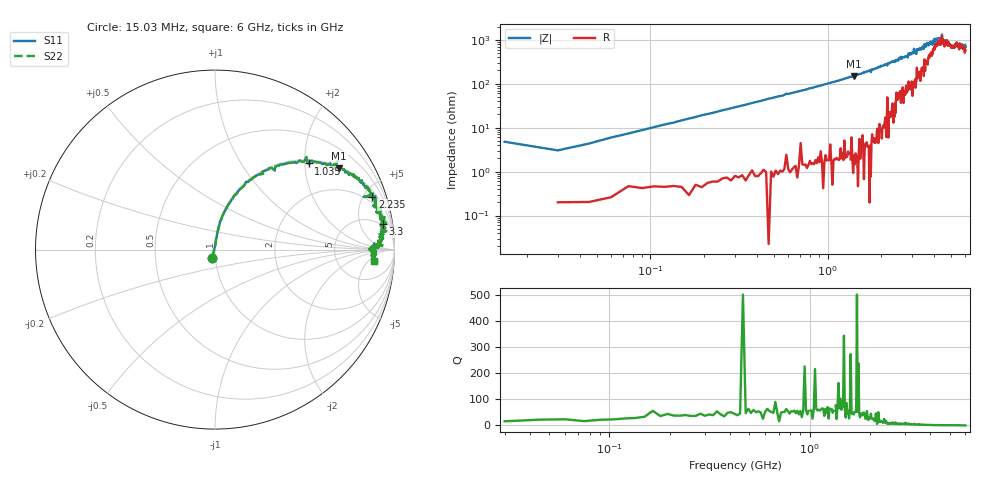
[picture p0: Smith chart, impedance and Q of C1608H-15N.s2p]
!	Network	Analyzer	HP8753E.07.74:	Oct	30	2002	Serial	No.	JP38451487
!	Hewlett-Packard
!	7	Sep	2009	10:19:27
!	Frequency	S11	S21	S12	S22
#	HZ	S	RI	R	50
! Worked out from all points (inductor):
!   400 points, 15.03 MHz to 6 GHz, reference 50 ohm
!   read as one part in series: L = 15.6 nH near 45.03 MHz
!   highest Q = 72 at 1.41 GHz (marker M1), where L = 17 nH
!   self-resonance near 4.927 GHz
!   S11 on the Smith chart (normalised r, x): 15.03 MHz: 0.96, -0.09; 1.035 GHz: 1.08, +2.09; 2.235 GHz: 1.45, +5.79; 3.3 GHz: 4, +12; 6 GHz: 12, -8
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1.502992e7  -0.016 -0.0452  1.02 0.0452  1.02 0.0452  -0.016 -0.0452
3.002985e7  0.00283 0.0302  0.997 -0.0302  0.997 -0.0302  0.00283 0.0302
6.00297e7  0.00625 0.0591  0.994 -0.0591  0.994 -0.0591  0.00625 0.0591
1.200294e8  0.0179 0.115  0.982 -0.115  0.982 -0.115  0.0179 0.115
3.300284e8  0.099 0.286  0.901 -0.286  0.901 -0.286  0.099 0.286
1.020025e9  0.514 0.491  0.486 -0.491  0.486 -0.491  0.514 0.491
1.035025e9  0.522 0.48  0.478 -0.48  0.478 -0.48  0.522 0.48
1.410023e9  0.692 0.454  0.308 -0.454  0.308 -0.454  0.692 0.454
2.01002e9  0.852 0.337  0.148 -0.337  0.148 -0.337  0.852 0.337
2.235019e9  0.876 0.293  0.124 -0.293  0.124 -0.293  0.876 0.293
3.015015e9  0.945 0.181  0.0546 -0.181  0.0546 -0.181  0.945 0.181
3.300014e9  0.936 0.141  0.0636 -0.141  0.0636 -0.141  0.936 0.141
3.91501e9  0.917 0.0865  0.0833 -0.0865  0.0833 -0.0865  0.917 0.0865
4.00501e9  0.936 0.0628  0.0637 -0.0628  0.0637 -0.0628  0.936 0.0628
4.365008e9  0.909 0.0467  0.0914 -0.0467  0.0914 -0.0467  0.909 0.0467
4.425008e9  0.933 0.0237  0.0667 -0.0237  0.0667 -0.0237  0.933 0.0237
4.455008e9  0.901 0.031  0.0991 -0.031  0.0991 -0.031  0.901 0.031
4.575007e9  0.886 0.0345  0.114 -0.0345  0.114 -0.0345  0.886 0.0345
4.725006e9  0.908 0.00922  0.0921 -0.00922  0.0921 -0.00922  0.908 0.00922
5.010005e9  0.874 0.00259  0.126 -0.00259  0.126 -0.00259  0.874 0.00259
5.355003e9  0.898 -0.0128  0.102 0.0128  0.102 0.0128  0.898 -0.0128
6e9  0.887 -0.0643  0.113 0.0643  0.113 0.0643  0.887 -0.0643
